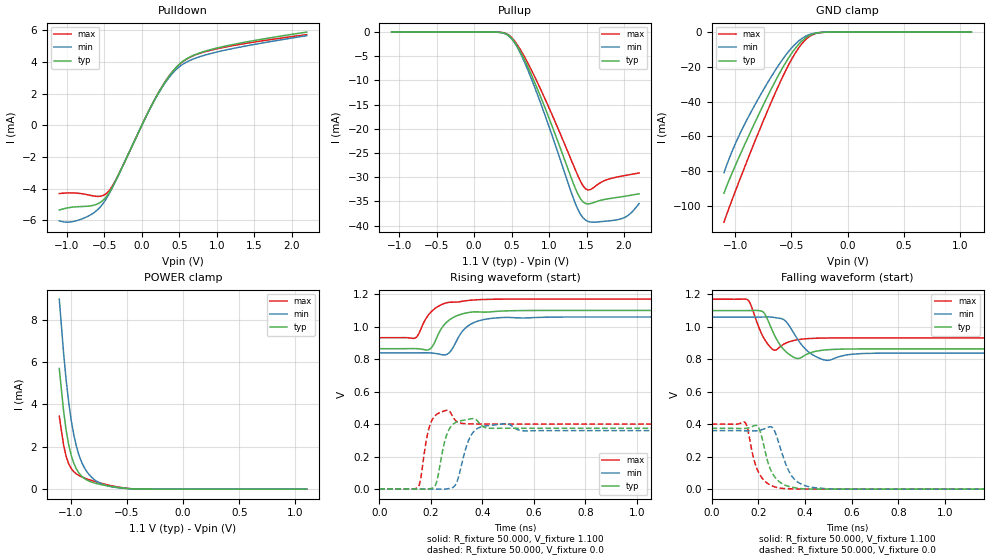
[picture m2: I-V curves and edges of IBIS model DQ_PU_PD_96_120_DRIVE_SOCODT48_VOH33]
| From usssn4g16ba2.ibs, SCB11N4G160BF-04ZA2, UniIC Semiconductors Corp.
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|   Model DQ_PU_PD_96_120_DRIVE_SOCODT48_VOH33
[Model] DQ_PU_PD_96_120_DRIVE_SOCODT48_VOH33
Model_type I/O
Polarity   Inverting
Vinl =  98.000mV
Vinh =  0.268V
Vmeas =  0.183V
Rref =  50.000
Vref =  0.183V
C_comp   1.020pF   1.010pF   1.030pF
[Model Spec]
Vinh   0.268V   0.262V   0.280V
Vinl   98.000mV   92.000mV   0.110V
Vmeas   0.183V   0.177V   0.195V
Vref   0.183V   0.177V   0.195V
Rref   50.000   NA   NA
[Temperature Range]   25.000   0.105k   -40.000
[Voltage Range]   1.100V   1.060V   1.170V
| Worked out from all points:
|   slope of the pulldown table from 0 to 0.165 V, typ, clamps not added: 105 ohm
|   GND clamp passes 1 mA (typ) near -0.30 V on its own axis
|   POWER clamp passes 1 mA (typ) near -0.95 V on its own axis
|   rising waveform, R_fixture 50.000, V_fixture 1.100: 20-80 % time 65.9ps typ, 65.2ps min, 65.9ps max; typ from 0.864 V to 1.1 V
|   rising waveform, R_fixture 50.000, V_fixture 0.0: 20-80 % time 27.9ps typ, 36.6ps min, 22.7ps max; typ from 0 V to 0.374 V
|   falling waveform, R_fixture 50.000, V_fixture 1.100: 20-80 % time 45.9ps typ, 61.1ps min, 35.7ps max; typ from 1.1 V to 0.864 V
|   falling waveform, R_fixture 50.000, V_fixture 0.0: 20-80 % time 51.8ps typ, 61.2ps min, 48.7ps max; typ from 0.374 V to 0 V
[Pulldown]
|Voltage   I(typ)   I(min)   I(max)
-1.1V     -5.34mA    -6.026mA   -4.302mA
-930mV    -5.164mA   -6.082mA   -4.26mA
-726mV    -5.101mA   -5.754mA   -4.373mA
-556mV    -4.87mA    -5.165mA   -4.475mA
-454mV    -4.386mA   -4.479mA   -4.222mA
-318mV    -3.209mA   -3.211mA   -3.18mA
192mV     1.799mA    1.766mA    1.806mA
362mV     3.096mA    3.011mA    3.096mA
532mV     3.983mA    3.811mA    3.973mA
702mV     4.448mA    4.219mA    4.427mA
1.008V    4.891mA    4.64mA     4.842mA
2.2V      5.891mA    5.665mA    5.73mA
[Pullup]
|Voltage   I(typ)   I(min)   I(max)
-1.1V     2.6nA      27.46nA    0A
432mV     -421.9uA   -476.8uA   -329.3uA
568mV     -2.729mA   -2.923mA   -2.437mA
704mV     -6.762mA   -7.352mA   -6.026mA
942mV     -15.5mA    -17.03mA   -13.67mA
1.316V    -30.95mA   -34mA      -27.19mA
1.452V    -35.08mA   -38.36mA   -31.74mA
1.554V    -35.42mA   -39.25mA   -32.53mA
1.724V    -34.63mA   -39.11mA   -30.79mA
1.928V    -34.12mA   -38.72mA   -29.88mA
2.064V    -33.78mA   -37.75mA   -29.49mA
2.2V      -33.41mA   -35.44mA   -29.11mA
[GND_clamp]
|Voltage   I(typ)   I(min)   I(max)
-1.1V     -92.78mA   -81.05mA   -109.5mA
-1.031V   -81.73mA   -69.22mA   -97.17mA
-939mV    -68.18mA   -56.02mA   -81.64mA
-824mV    -52mA      -41.83mA   -62.83mA
-686mV    -33.62mA   -26.41mA   -41.32mA
-571mV    -19.76mA   -15.06mA   -24.85mA
-479mV    -10.5mA    -7.76mA    -13.5mA
-410mV    -5.313mA   -3.84mA    -6.916mA
-341mV    -2.007mA   -1.45mA    -2.59mA
-272mV    -506.9uA   -403.5uA   -609.8uA
-180mV    -45.65uA   -51.35uA   -43.55uA
1.1V      0A         0A         0A
[POWER_clamp]
|Voltage   I(typ)   I(min)   I(max)
-1.1V     5.691mA    8.967mA    3.44mA
-1.062V   3.709mA    6.444mA    2.092mA
-1.039V   2.781mA    5.152mA    1.546mA
-1.016V   2.086mA    4.085mA    1.193mA
-970mV    1.21mA     2.539mA    818.5uA
-947mV    943.7uA    2.005mA    716.7uA
-901mV    610.1uA    1.27mA     581.3uA
-855mV    430.7uA    824.1uA    484.6uA
-786mV    289.9uA    439.4uA    366uA
-671mV    155.9uA    155.9uA    203.6uA
-441mV    13.2uA     12.79uA    15.03uA
1.1V      0A         0A         0A
[Ramp]
| variable   typ   min   max
dV/dt_r   0.225/28.071p   0.216/36.890p   0.240/22.829p
dV/dt_f   0.141/46.030p   0.133/61.069p   0.143/35.833p
R_load = 50.000
[Rising Waveform]
R_fixture= 50.000
V_fixture= 1.100
V_fixture_min= 1.060
V_fixture_max= 1.170
|time   V(typ)   V(min)   V(max)
0s        864.4mV    838.5mV    932.1mV
140ps     864.9mV    838.7mV    930.6mV
195ps     860.3mV    838.7mV    1.08V
262ps     1.028V     829.2mV    1.147V
280ps     1.05V      855.5mV    1.151V
331ps     1.082V     986.3mV    1.158V
385ps     1.091V     1.035V     1.166V
479ps     1.096V     1.056V     1.169V
726ps     1.1V       1.06V      1.17V
3ns       1.1V       1.06V      1.17V
[Rising Waveform]
R_fixture= 50.000
V_fixture= 0.0
V_fixture_min= 0.0
V_fixture_max= 0.0
|time   V(typ)   V(min)   V(max)
0s        4.356uV    15.89uV    1.031uV
150ps     -230.3uV   73.1uV     10.2mV
198ps     2.53mV     -168uV     399.7mV
223ps     45.96mV    -391.4uV   459.9mV
261ps     330.7mV    830.3uV    485.2mV
299ps     411.9mV    35.5mV     418.1mV
364ps     434mV      349.1mV    400.9mV
489ps     374.4mV    402.7mV    400.4mV
567ps     374.4mV    358.2mV    400.4mV
3ns       374.4mV    360.1mV    400.4mV
[Falling Waveform]
R_fixture= 50.000
V_fixture= 1.100
V_fixture_min= 1.060
V_fixture_max= 1.170
|time   V(typ)   V(min)   V(max)
0s        1.1V       1.06V      1.17V
157ps     1.1V       1.06V      1.164V
222ps     1.09V      1.061V     935.8mV
272ps     941.6mV    1.057V     856mV
315ps     851.7mV    1.038V     897.4mV
362ps     806.3mV    938.3mV    918.7mV
420ps     838.4mV    840.3mV    928mV
496ps     858.7mV    793.2mV    931.2mV
700ps     864.3mV    837.3mV    932.1mV
3ns       864.4mV    838.5mV    932.1mV
[Falling Waveform]
R_fixture= 50.000
V_fixture= 0.0
V_fixture_min= 0.0
V_fixture_max= 0.0
|time   V(typ)   V(min)   V(max)
0s        374.4mV    360.1mV    400.4mV
143ps     373.6mV    359.5mV    411.3mV
154ps     376mV      359.2mV    373.3mV
196ps     389.5mV    360.2mV    119.8mV
262ps     94.18mV    376.9mV    18.76mV
299ps     36.2mV     233.1mV    4.981mV
330ps     16.65mV    114mV      2.278mV
368ps     5.906mV    44.68mV    870.6uV
508ps     107.8uV    1.213mV    24.52uV
3ns       4.347uV    15.86uV    1.092uV
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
